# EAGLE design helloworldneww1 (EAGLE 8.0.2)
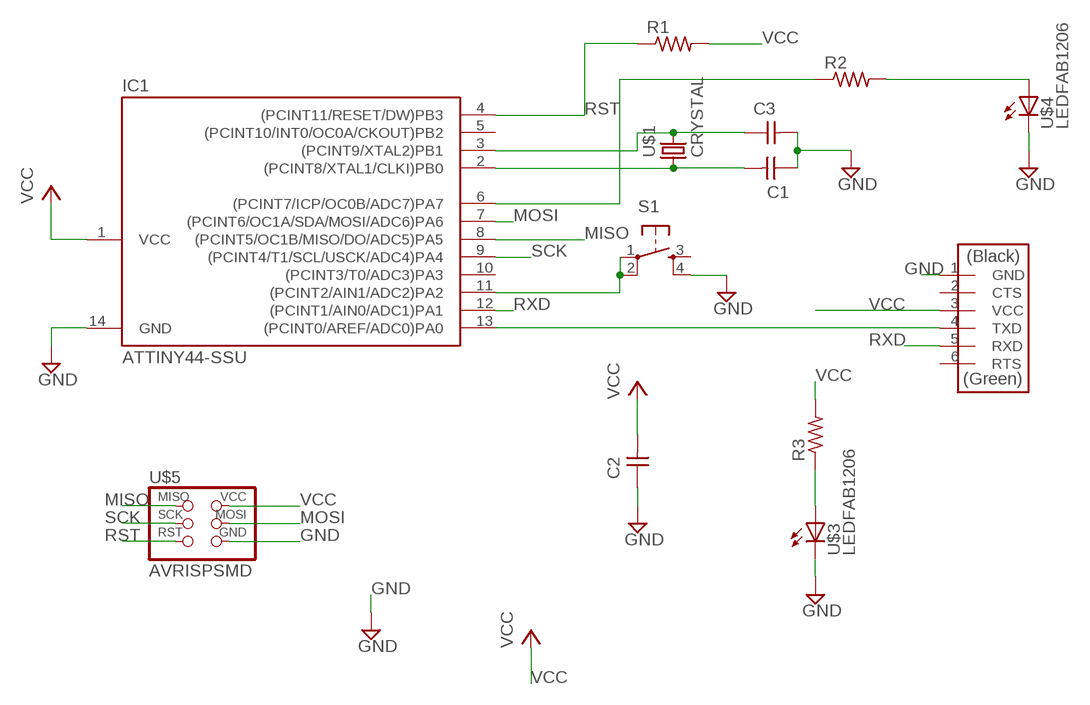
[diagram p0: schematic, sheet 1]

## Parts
C1  CAP-UNPOLARIZEDFAB  [C1206FAB]
C2  CAP-UNPOLARIZEDFAB  [C1206FAB]
C3  CAP-UNPOLARIZEDFAB  [C1206FAB]
IC1  ATTINY44-SSU  [SOIC14]
R1  RES-US1206FAB  [R1206FAB]
R2  RES-US1206FAB  [R1206FAB]
R3  RES-US1206FAB  [R1206FAB]
S1  6MM_SWITCH6MM_SWITCH  [6MM_SWITCH]
U$1  CRYSTAL  [2-SMD-5X3MM]
U$2  FTDI-SMD-HEADER  [1X06SMD]
U$3  LEDFAB1206  [LED1206FAB]
U$4  LEDFAB1206  [LED1206FAB]
U$5  AVRISPSMD  [2X03SMD]

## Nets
GND: C1.1 C2.1 C3.2 IC1.14(GND) S1.4(S1) U$2.1(GND) U$3.2(C) U$4.2(C) U$5.6(GND)
MISO: IC1.8((PCINT5/OC1B/MISO/DO/ADC5)PA5) U$5.1(MISO)
MOSI: IC1.7((PCINT6/OC1A/SDA/MOSI/ADC6)PA6) U$5.4(MOSI)
N$1: IC1.13((PCINT0/AREF/ADC0)PA0) U$2.4(TXD)
N$2: C3.1 IC1.3((PCINT9/XTAL2)PB1) U$1.P$2
N$3: C1.2 IC1.2((PCINT8/XTAL1/CLKI)PB0) U$1.P$1
N$4: IC1.6((PCINT7/ICP/OC0B/ADC7)PA7) R2.1
N$5: R2.2 U$4.1(A)
N$6: R3.1 U$3.1(A)
N$7: IC1.11((PCINT2/AIN1/ADC2)PA2) S1.1(P) S1.2(P1)
RST: IC1.4((PCINT11/RESET/DW)PB3) R1.1 U$5.5(RST)
RXD: IC1.12((PCINT1/AIN0/ADC1)PA1) U$2.5(RXD)
SCK: IC1.9((PCINT4/T1/SCL/USCK/ADC4)PA4) U$5.3(SCK)
VCC: C2.2 IC1.1(VCC) R1.2 R3.2 U$2.3(VCC) U$5.2(VCC)
Unconnected: IC1.5((PCINT10/INT0/OC0A/CKOUT)PB2) IC1.10((PCINT3/T0/ADC3)PA3) S1.3(S) U$2.2(CTS) U$2.6(RTS)

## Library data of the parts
C1-C3 = fab:CAP-UNPOLARIZED
IC1 = fab:ATTINY44
R1-R3 = fab:RES-US: Resistor (US Symbol)
S1 = fab:6MM_SWITCH: OMRON SWITCH
U$1 = fab:CRYSTAL
U$2 = fab:FTDI-SMD-HEADER
U$3 U$4 = fab:LED: LED
U$5 = fab:AVRISP

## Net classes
0 default: clearance 0.205 mm

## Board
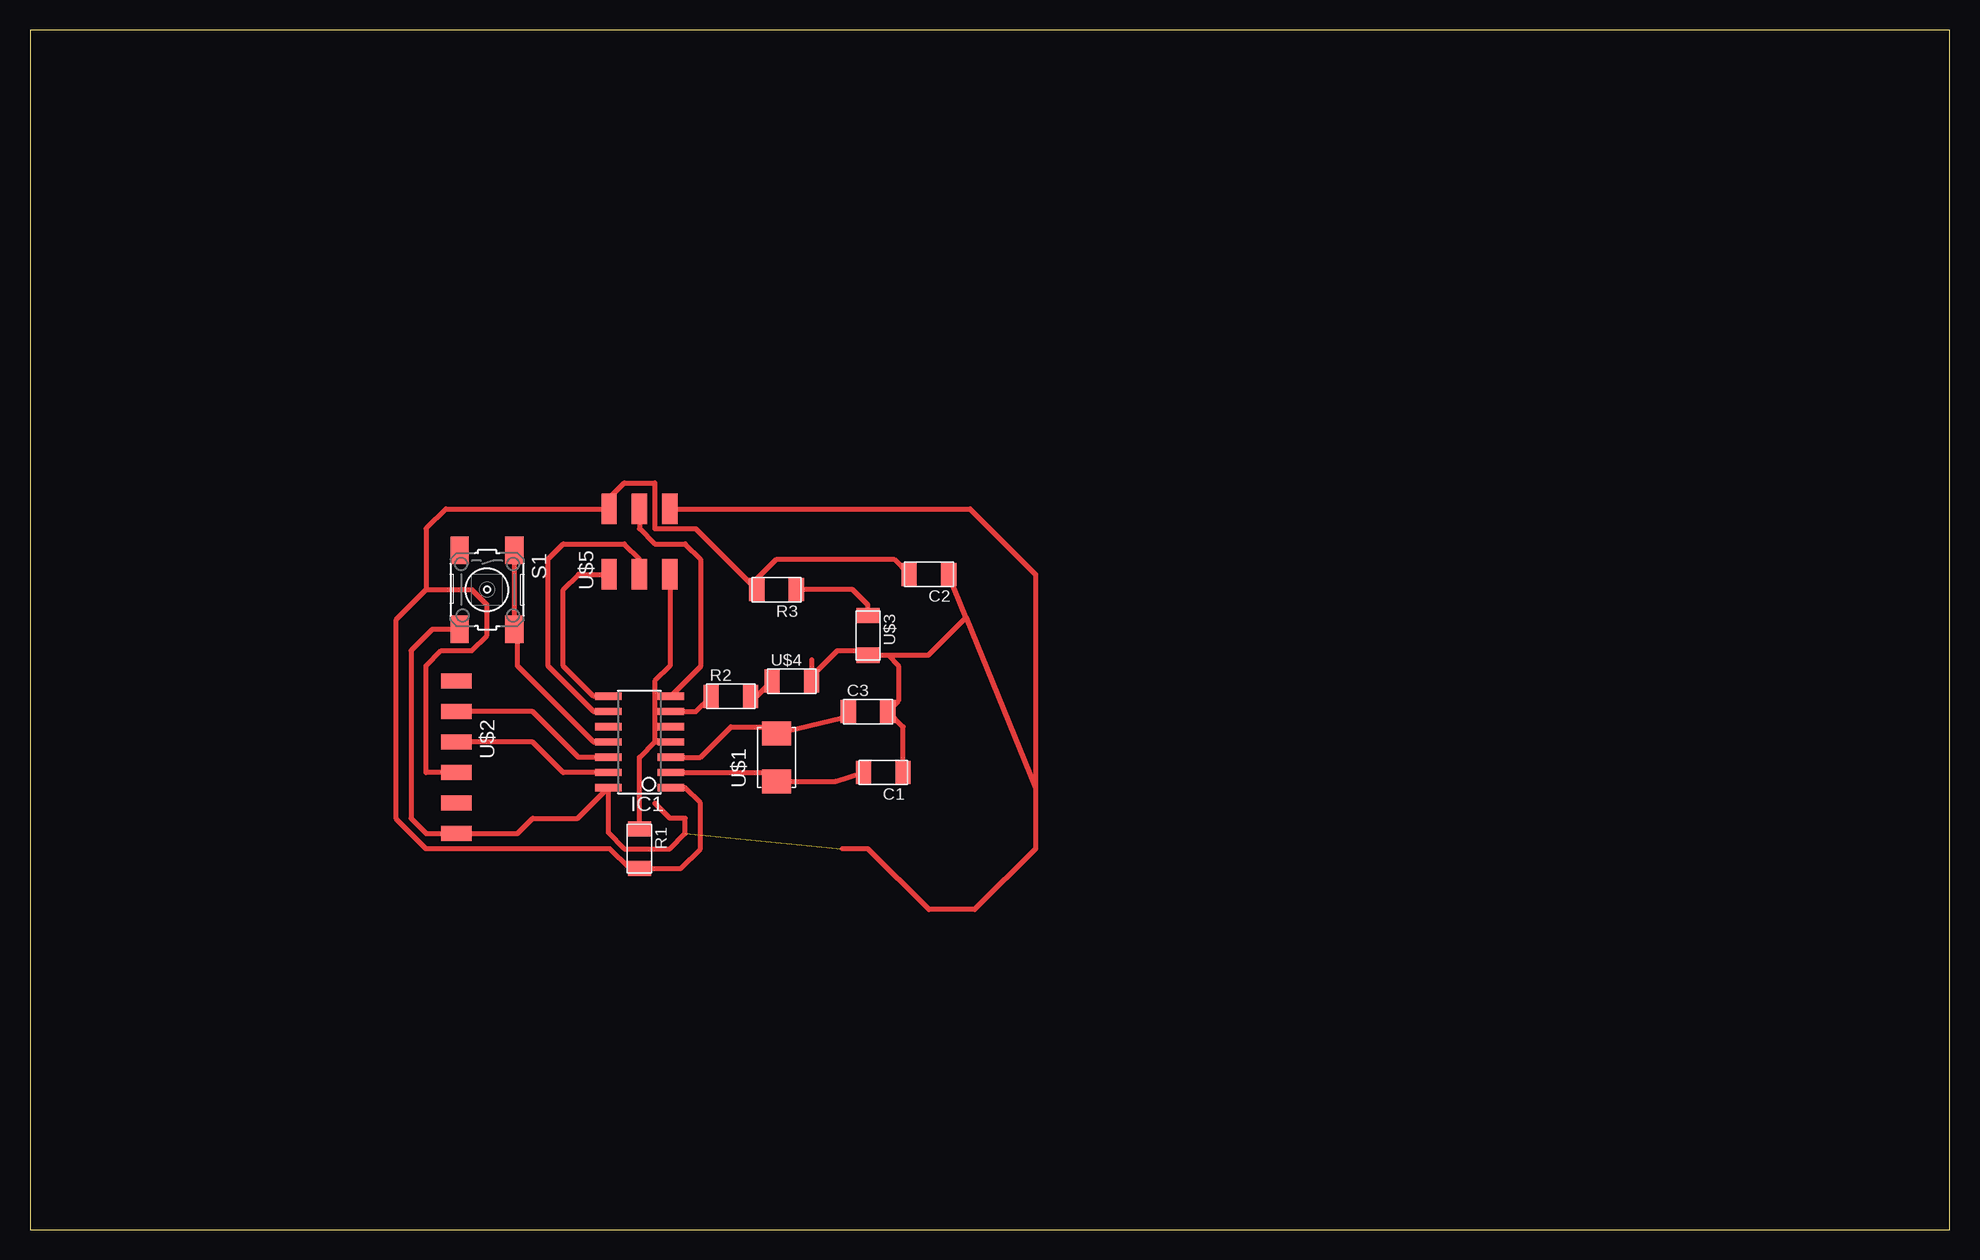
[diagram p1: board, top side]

Size 160 x 100 mm. Coordinates in mm from the lower left corner, seen from the top.
Outline: 0,0 160,0 160,100 0,100 0,0
Copper layers (1*16): Top 0.035mm / dielectric 1.5mm / Bottom 0.035mm
Design rules "default": minimum track width 10mil, minimum drill 24mil, track to track 8mil, track to pad 8mil, pad to pad 8mil, via to via 8mil, smd to smd 8mil, copper to edge 40mil, drill to drill 8mil, minimum pad ring 10mil, minimum via ring 8mil, stop-mask expansion 4mil, vias tented up to drill 0mil, thermal gap 10mil

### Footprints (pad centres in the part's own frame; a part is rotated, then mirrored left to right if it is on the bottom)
C1206FAB = smd 1.27 x 1.905: 1 -1.651,0; 2 1.651,0
SOIC14 = smd 0.61 x 2.21: 1 -3.81,-2.603; 2 -2.54,-2.603; 3 -1.27,-2.603; 4 0,-2.603; 5 1.27,-2.603; 6 2.54,-2.603; 7 3.81,-2.603; 8 3.81,2.603; 9 2.54,2.603; 10 1.27,2.603; 11 0,2.603; 12 -1.27,2.603; 13 -2.54,2.603; 14 -3.81,2.603
R1206FAB = smd 1.27 x 1.905: 1 -1.651,0; 2 1.651,0
6MM_SWITCH = smd 2.286 x 1.524: 1 -3.302,2.286; 2 3.302,2.286; 3 -3.302,-2.286; 4 3.302,-2.286
2-SMD-5X3MM = smd 2 x 2.4: P$1 -2,0; P$2 2,0
1X06SMD = smd 2.54 x 1.27: 1 0,6.35; 2 0,3.81; 3 0,1.27; 4 0,-1.27; 5 0,-3.81; 6 0,-6.35
LED1206FAB = smd 1.27 x 1.905: 1 -1.651,0; 2 1.651,0
2X03SMD = smd 2.54 x 1.27: 1 -2.54,2.54; 2 2.92,2.54; 3 -2.54,0; 4 2.92,0; 5 -2.54,-2.54; 6 2.92,-2.54

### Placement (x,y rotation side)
C1  71.12,38.1 180 top
C2  74.93,54.61 180 top
C3  69.85,43.18 0 top
IC1  50.8,40.64 90 top
R1  50.8,31.75 270 top
R2  58.42,44.45 0 top
R3  62.23,53.34 180 top
S1  38.1,53.34 270 top
U$1  62.23,39.37 90 top
U$2  35.56,39.37 180 top
U$3  69.85,49.53 270 top
U$4  63.5,45.72 0 top
U$5  50.8,57.15 90 top

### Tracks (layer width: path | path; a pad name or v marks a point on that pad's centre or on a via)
GND  (1 unrouted)
  Top 0.406: S1.4 33.53,50.04 31.75,48.26 31.75,34.29 33.02,33.02 U$2.1 40.64,33.02 41.91,34.29 45.66,34.29 IC1.14 48.2,33.08 49.53,31.75 53.34,31.75 54.61,33.02 54.61,34.29 53.34,34.29 52.07,35.56 | U$5.6 78.36,60.07 83.82,54.61 83.82,36.83 | 83.82,36.83 83.82,31.75 78.74,26.67 74.93,26.67 69.85,31.75 67.69,31.75 | 78.04,51.03 C2.1 | 78.04,51.03 83.82,36.83 | U$3.2 71.5,47.88 72.39,46.99 72.39,44.07 C3.2 72.77,41.91 C1.1 | 65.15,47.5 U$4.2 65.15,46.1 67.31,48.26 69.47,48.26 U$3.2 | U$3.2 74.89,47.88 78.04,51.03
MISO
  Top 0.406: IC1.8 46.99,44.45 44.45,46.99 44.45,53.34 45.72,54.61 U$5.1
MOSI
  Top 0.406: U$5.4 50.8,58.42 52.07,57.15 54.61,57.15 55.88,55.88 55.88,46.93 IC1.7
N$1
  Top 0.406: IC1.13 44.45,38.1 41.91,40.64 U$2.4
N$2
  Top 0.406: IC1.3 55.88,39.37 58.42,41.91 61.5,41.91 U$1.P$2 67.66,42.64 C3.1
N$3
  Top 0.406: IC1.2 61.69,38.1 U$1.P$1 67.15,37.37 C1.2
N$4
  Top 0.406: IC1.6 55.5,43.18 R2.1
N$5
  Top 0.406: R2.2 60.58,44.45 U$4.1
N$6
  Top 0.406: U$3.1 69.85,52.07 68.58,53.34 R3.1
N$7
  Top 0.406: IC1.11 46.99,40.64 40.64,46.99 40.64,49.78 S1.2 S1.1
RST
  Top 0.406: 51.18,33.4 R1.1 50.8,39.37 52.07,40.64 | 52.07,40.64 IC1.4 | U$5.5 53.34,46.99 52.07,45.72 52.07,40.64
RXD
  Top 0.406: IC1.12 45.72,39.37 41.91,43.18 U$2.5
SCK
  Top 0.406: IC1.9 46.99,43.18 43.18,46.99 43.18,55.88 44.45,57.15 49.53,57.15 50.8,55.88 U$5.3
VCC
  Top 0.406: U$2.3 33.02,38.1 33.02,46.99 34.29,48.26 36.83,48.26 38.1,49.53 38.1,52.07 36.83,53.34 33.02,53.34 | 33.02,53.34 30.48,50.8 30.48,34.29 33.02,31.75 48.32,31.75 49.97,30.1 R1.2 | 33.02,53.34 33.02,58.42 34.67,60.07 U$5.2 48.26,60.96 49.53,62.23 52.07,62.23 52.07,58.42 55.5,58.42 R3.2 60.58,54.23 62.23,55.88 72.01,55.88 C2.2 | R1.2 51.69,30.1 | 53.34,36.77 IC1.1 54.61,36.83 55.88,35.56 55.88,31.75 54.23,30.1 R1.2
